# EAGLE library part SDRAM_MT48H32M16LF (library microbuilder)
MT48H32M16LF - Mobile Low-Power SDR SDRAM 512MBits (8 Meg x 16 x 4 banks) 1.8V, 133MHz, -40°C-85°C Digikey: 557-1389-1-ND
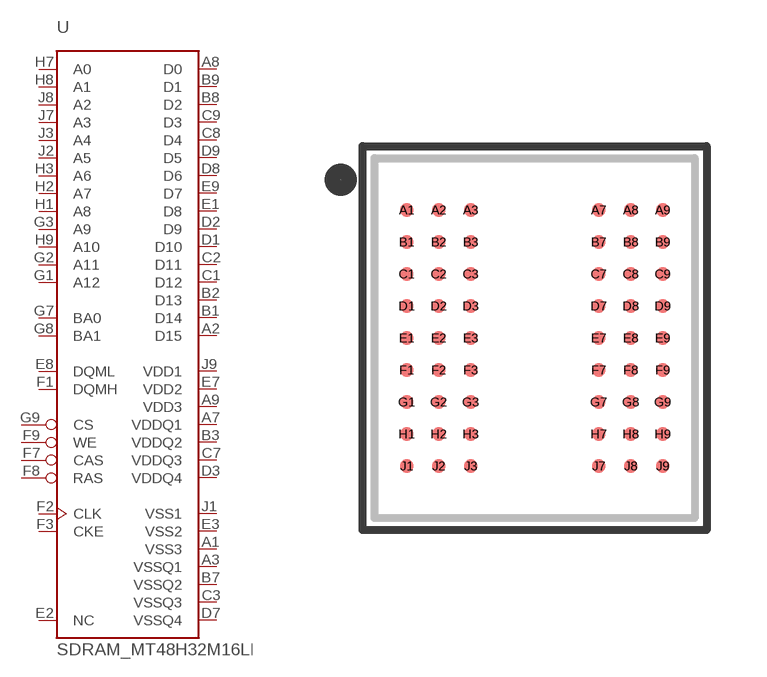
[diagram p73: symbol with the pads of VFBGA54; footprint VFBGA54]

Designator prefix U

## SDRAM_MT48H32M16LF  [VFBGA54]
A1  VSS3
A2  D15
A3  VSSQ1
A7  VDDQ1
A8  D0
A9  VDD3
B1  D14
B2  D13
B3  VDDQ2
B7  VSSQ2
B8  D2
B9  D1
C1  D12
C2  D11
C3  VSSQ3
C7  VDDQ3
C8  D4
C9  D3
D1  D10
D2  D9
D3  VDDQ4
D7  VSSQ4
D8  D6
D9  D5
E1  D8
E2  NC
E3  VSS2
E7  VDD2
E8  DQML
E9  D7
F1  DQMH
F2  CLK
F3  CKE
F7  CAS
F8  RAS
F9  WE
G1  A12
G2  A11
G3  A9
G7  BA0
G8  BA1
G9  CS
H1  A8
H2  A7
H3  A6
H7  A0
H8  A1
H9  A10
J1  VSS1
J2  A5
J3  A4
J7  A3
J8  A2
J9  VDD1

## Footprint VFBGA54 (pad centres in mm)
vFBGA180 (8mm x 9mm, 0.8mm pitch, 0.45mm balls) Source: http://download.micron.com/pdf/datasheets/dram/mobile/512mb_mobile_sdram_y47m.pdf Pad size is 0.34mm copper and ~0.5mm total with the solder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
smd 0.34 x 0.34: A1 -3.2,3.2; A2 -2.4,3.2; A3 -1.6,3.2; A7 1.6,3.2; A8 2.4,3.2; A9 3.2,3.2; B1 -3.2,2.4; B2 -2.4,2.4; B3 -1.6,2.4; B7 1.6,2.4; B8 2.4,2.4; B9 3.2,2.4; C1 -3.2,1.6; C2 -2.4,1.6; C3 -1.6,1.6; C7 1.6,1.6; C8 2.4,1.6; C9 3.2,1.6; D1 -3.2,0.8; D2 -2.4,0.8; D3 -1.6,0.8; D7 1.6,0.8; D8 2.4,0.8; D9 3.2,0.8; E1 -3.2,0; E2 -2.4,0; E3 -1.6,0; E7 1.6,0; E8 2.4,0; E9 3.2,0; F1 -3.2,-0.8; F2 -2.4,-0.8; F3 -1.6,-0.8; F7 1.6,-0.8; F8 2.4,-0.8; F9 3.2,-0.8; G1 -3.2,-1.6; G2 -2.4,-1.6; G3 -1.6,-1.6; G7 1.6,-1.6; G8 2.4,-1.6; G9 3.2,-1.6; H1 -3.2,-2.4; H2 -2.4,-2.4; H3 -1.6,-2.4; H7 1.6,-2.4; H8 2.4,-2.4; H9 3.2,-2.4; J1 -3.2,-3.2; J2 -2.4,-3.2; J3 -1.6,-3.2; J7 1.6,-3.2; J8 2.4,-3.2; J9 3.2,-3.2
